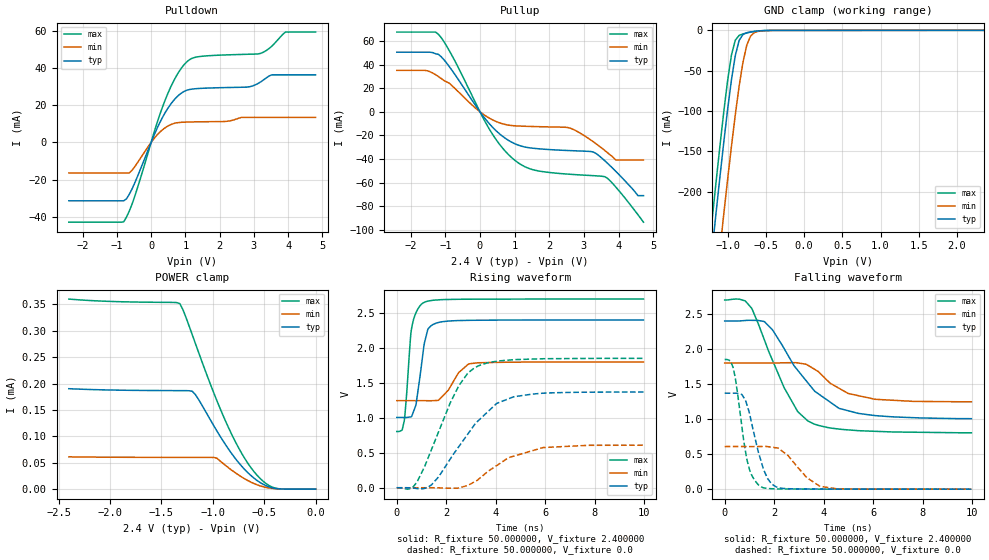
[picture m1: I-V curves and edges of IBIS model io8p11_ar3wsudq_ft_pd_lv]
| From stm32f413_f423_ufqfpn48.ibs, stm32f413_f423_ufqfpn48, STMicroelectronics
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|   Model io8p11_ar3wsudq_ft_pd_lv
[Model]  io8p11_ar3wsudq_ft_pd_lv
Model_type I/O
Polarity   Non-Inverting
Enable   Active-Low
Vinl =   0.720000V
Vinh =   1.680000V
Vmeas =  1.200000V
Cref =   30.000000pF
Rref =   100.000000M
Vref =   0.0V
C_comp   3.740800pF   3.684200pF   3.822900pF
[Temperature Range]   25.000000   0.125000k   -40.000000
[Pullup Reference]   2.400000V   1.800000V   2.700000V
[Pulldown Reference]   0.0V   0.0V   0.0V
[POWER Clamp Reference]   2.400000V   1.800000V   2.700000V
[GND Clamp Reference]   0.0V   0.0V   0.0V
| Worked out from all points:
|   slope of the pulldown table from 0 to 0.36 V, typ, clamps not added: 25 ohm
|   slope of the pullup table from 0 to 0.36 V, typ, clamps not added: 27.7 ohm
|   GND clamp passes 1 mA (typ) near -0.62 V on its own axis
|   rising waveform, R_fixture 50.000000, V_fixture 2.400000: 20-80 % time 337ps typ, 660ps min, 257ps max; typ from 1 V to 2.4 V
|   rising waveform, R_fixture 50.000000, V_fixture 0.0: 20-80 % time 1.79ns typ, 1.76ns min, 1.35ns max; typ from 0 V to 1.37 V
|   falling waveform, R_fixture 50.000000, V_fixture 2.400000: 20-80 % time 1.89ns typ, 1.37ns min, 1.43ns max; typ from 2.4 V to 1 V
|   falling waveform, R_fixture 50.000000, V_fixture 0.0: 20-80 % time 587ps typ, 967ps min, 463ps max; typ from 1.37 V to 0 V
[Pulldown]
|Voltage   I(typ)   I(min)   I(max)
-2.4V     -31.47mA   -16.45mA   -43.01mA
-800mV    -31.47mA   -16.45mA   -42.85mA
-480mV    -21.98mA   -13.17mA   -29.2mA
80mV      3.63mA     1.966mA    5.014mA
480mV     18.15mA    8.738mA    26.02mA
800mV     25.38mA    10.72mA    37.77mA
1.12V     28.53mA    11.02mA    44.6mA
2.8V      29.84mA    13.51mA    47.53mA
3.2V      32.66mA    13.51mA    48.04mA
3.52V     36.44mA    13.51mA    51.84mA
3.92V     36.44mA    13.51mA    59.49mA
4.8V      36.44mA    13.51mA    59.49mA
[Pullup]
|Voltage   I(typ)   I(min)   I(max)
-2.4V     50.45mA    35.08mA    67.51mA
-1.52V    50.45mA    34.74mA    67.51mA
-1.2V     48.64mA    29.87mA    65.66mA
320mV     -11.75mA   -6.207mA   -17.08mA
1.04V     -27.54mA   -11.97mA   -41.91mA
1.6V      -31.13mA   -12.58mA   -49.63mA
2.56V     -32.88mA   -13.52mA   -52.9mA
3.28V     -34.25mA   -25.63mA   -54.18mA
3.6V      -41.44mA   -32.74mA   -55.03mA
3.92V     -50.47mA   -40.9mA    -63.79mA
4.56V     -71.1mA    -40.9mA    -87.26mA
4.72V     -71.1mA    -40.9mA    -93.6mA
[GND_clamp]
|Voltage   I(typ)   I(min)   I(max)
-2.4V     -1.429A    -1.514A    -1.398A
-1.25V    -315.9mA   -407.2mA   -278.2mA
-1.2V     -270.1mA   -361.3mA   -232.1mA
-1.15V    -225mA     -316mA     -186.8mA
-1.1V     -180.9mA   -271.3mA   -142.7mA
-1.05V    -138.2mA   -227.5mA   -100.5mA
-950mV    -61.14mA   -143.6mA   -30.44mA
-900mV    -31.24mA   -104.7mA   -12.15mA
-850mV    -12.5mA    -69.41mA   -6.236mA
-750mV    -2.91mA    -18.35mA   -3.195mA
-600mV    -761.5uA   -1.227mA   -751.9uA
2.35V     58.09uA    37.93uA    67.25uA
[POWER_clamp]
|Voltage   I(typ)   I(min)   I(max)
-2.4V     190.2uA    61.19uA    359.9uA
-1.32V    186.6uA    60.14uA    351.2uA
-1.29V    186.5uA    60.13uA    339.6uA
-1.2V     185.4uA    60.11uA    292.6uA
-1.17V    179.2uA    60.11uA    276.3uA
-960mV    110.2uA    58.62uA    167.5uA
-870mV    82.44uA    43.99uA    126.3uA
-750mV    50.58uA    26.92uA    78.64uA
-630mV    25.94uA    13.41uA    41.02uA
-510mV    9.22uA     4.527uA    14.97uA
-420mV    2.425uA    1.38uA     3.75uA
0V        0A         0A         0A
[Ramp]
| variable   typ   min   max
dV/dt_r  0.82110/1.79267n   0.36358/1.74680n   1.11042/1.34598n
dV/dt_f  0.83310/1.88497n   0.33270/1.39339n   1.13542/1.42624n
R_load = 50.000000
[Rising Waveform]
R_fixture= 50.000000
V_fixture= 2.400000
V_fixture_min= 1.800000
V_fixture_max= 2.700000
|time   V(typ)   V(min)   V(max)
0s        1.005V     1.245V     804.3mV
220.2ps   1.005V     1.245V     829.3mV
320.3ps   1.005V     1.246V     1V
600.6ps   1.019V     1.246V     2.282V
780.8ps   1.197V     1.246V     2.506V
1.081ns   1.987V     1.245V     2.646V
1.381ns   2.316V     1.244V     2.677V
1.682ns   2.363V     1.251V     2.687V
2.903ns   2.394V     1.771V     2.696V
9.97ns    2.399V     1.799V     2.698V
[Rising Waveform]
R_fixture= 50.000000
V_fixture= 0.0
V_fixture_min= 0.0
V_fixture_max= 0.0
|time   V(typ)   V(min)   V(max)
0s        164.8uV    65.13uV    284uV
820.8ps   -11.83mV   61.77uV    83.35mV
1.401ns   40.83mV    135.6uV    546.1mV
2.162ns   411.3mV    -6.863mV   1.216V
2.523ns   595.5mV    -1.309mV   1.467V
3.143ns   901.9mV    85.6mV     1.715V
4.044ns   1.207V     318.9mV    1.809V
4.725ns   1.3V       452.1mV    1.831V
5.926ns   1.352V     575.1mV    1.845V
9.97ns    1.369V     608.3mV    1.85V
[Falling Waveform]
R_fixture= 50.000000
V_fixture= 2.400000
V_fixture_min= 1.800000
V_fixture_max= 2.700000
|time   V(typ)   V(min)   V(max)
0s        2.399V     1.799V     2.698V
820.8ps   2.406V     1.799V     2.687V
1.101ns   2.409V     1.799V     2.574V
1.602ns   2.391V     1.799V     2.131V
2.402ns   2.005V     1.803V     1.448V
2.943ns   1.699V     1.801V     1.111V
3.363ns   1.516V     1.767V     972.8mV
4.605ns   1.157V     1.442V     857.9mV
5.405ns   1.08V      1.333V     834.3mV
9.97ns    1.005V     1.245V     804.3mV
[Falling Waveform]
R_fixture= 50.000000
V_fixture= 0.0
V_fixture_min= 0.0
V_fixture_max= 0.0
|time   V(typ)   V(min)   V(max)
0s        1.369V     608.3mV    1.85V
340.3ps   1.369V     608.4mV    1.733V
440.4ps   1.369V     608.4mV    1.56V
840.8ps   1.267V     608.2mV    539.9mV
1.081ns   954.5mV    608mV      207.8mV
1.441ns   433.1mV    608.5mV    38.53mV
1.722ns   160.9mV    607.4mV    10.32mV
2.042ns   39.95mV    591.7mV    4.803mV
3.864ns   1.599mV    39.39mV    1.005mV
9.97ns    164.8uV    65.13uV    284uV
